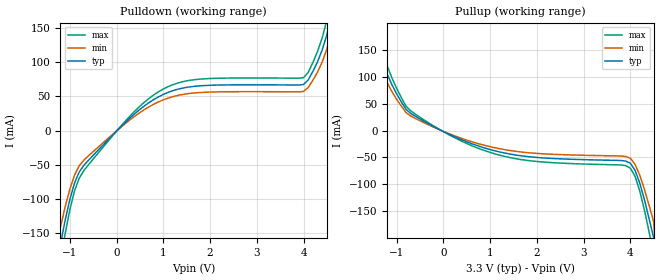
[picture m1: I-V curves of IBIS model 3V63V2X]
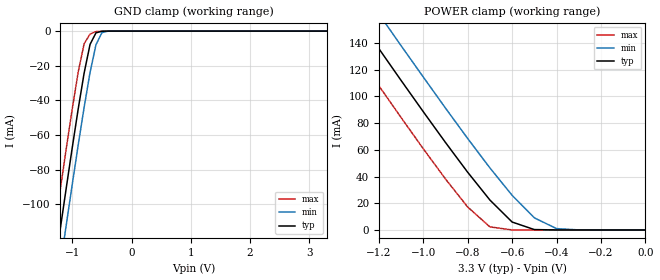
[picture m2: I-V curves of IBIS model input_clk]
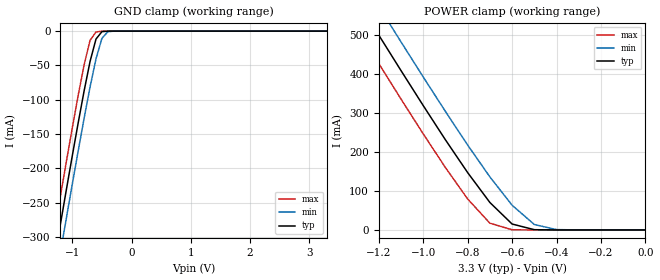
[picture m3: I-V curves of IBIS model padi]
[IBIS Ver]   2.1
[File name]   ics570-3.ibs
[File Rev]   3.0
[Date]   08/02/2010
[Source]   ICS MicroClock Applications Engineering 2
[Disclaimer] This information is for modeling purposes only, and is
(C) Copyright Integrated Circuit Systems, Inc. 1997-2001
   All rights reserved
ICS hereby grants the user of this IBIS model a non-exclusive,
nontransferable license to use this IBIS model under the following terms.
Before using this IBIS model, the user should read this license.
If the user does not accept these terms,  the IBIS model should be
returned to ICS within 30 days.
   The user is granted this license only to use the IBIS model and
is not granted rights to sell, load, rent, lease or license the IBIS
model in whole or in part, or in modified form to anyone other than
user. User may modify the IBIS model to suit its specific
applications but rights to derivative works and such modifications
shall belong to ICS.
   This IBIS model is provided on an "AS IS" basis and ICS makes
absolutely no warranty with respect to the information contained
herein. ICS DISCLAIMS AND CUSTOMER WAIVES ALL WARRANTIES, EXPRESS
OR IMPLIED, INCLUDING WARRANTIES OF MERCHANTABILITY OR FITNESS FOR
A PARTICULAR PURPOSE. The entire risk as to quality and performance
is with the Customer. ACCORDINGLY, IN NO EVENT SHALL THE COMPANY BE
LIABLE FOR ANY DAMAGES, WHETHER IN CONTRACT OR TORT,INCLUDING ANY
LOST PROFITS OR OTHER INCIDENTAL, CONSEQUENTIAL, EXEMPLARY, OR
PUNITIVE DAMAGES ARISING OUT OF THE USE OR APPLICATION OF THE IBIS
model provided in this package. Further, ICS reserves the right to
make changes without notice to any product herein to improve
reliability, function, or design. ICS does not convey any license
under patent rights or any other intellectual property rights,
including those of third parties.
   ICS is not obligated to provide maintenance or support
for the licensed IBIS model.
[Component]   ics570
[Manufacturer] Integrated Circuit Systems Inc.
[Package]
|   typ   min   max
R_pkg   40m   35m   45m
L_pkg   1.65nH   1.35nH   1.95nH
C_pkg   0.24pF   0.14pF   0.34pF
[pin]   signal_name   model_name   R_pin   L_pin   C_pin
4   ICLK   input_clk
5   FBIN   padi
7   CLK   3V63V2X
8   CLK/2   3V63V2X
| Models and submodels in the file (3): 3V63V2X (Output), input_clk (Input), padi (Input)
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|   ICS570 3.3V Clock Drive Model
| This model is suitable for all single output pins on the
| ICS570 FAMILY|
[Model]   3V63V2X
Model_type   Output
Polarity   Non-Inverting
|   typ   min   max
C_comp   5pF   4pF   6pF
|   typ   min   max
[Voltage range]  3.3V   3.15V   3.45V
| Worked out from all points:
|   slope of the pulldown table from 0 to 0.495 V, typ, clamps not added: 15.7 ohm
|   slope of the pullup table from 0 to 0.495 V, typ, clamps not added: 26.1 ohm
[pulldown]
|Voltage I (typ)   I (min)   I (max)
-3.3V     -3A        -3A        -3A
-1.3V     -199.9mA   -169.9mA   -229.9mA
-1.1V     -132mA     -112.2mA   -151.8mA
-900mV    -77.23mA   -65.65mA   -88.82mA
-700mV    -51.19mA   -43.51mA   -58.87mA
400mV     25.31mA    21.51mA    29.1mA
1.1V      55.9mA     47.52mA    64.28mA
4V        67.53mA    57.4mA     77.66mA
4.5V      140.8mA    119.7mA    161.9mA
4.6V      173.4mA    147.4mA    199.5mA
4.7V      200.4mA    170.3mA    230.4mA
6.6V      3A         3A         3A
[pullup]
|Voltage I (typ)   I (min)   I (max)
-3.3V     3A         3A         3A
-1.5V     200.3mA    170.3mA    230.4mA
-1.4V     161.7mA    137.4mA    185.9mA
-1.2V     103.9mA    88.33mA    119.5mA
-800mV    39.29mA    33.4mA     45.19mA
200mV     -10.06mA   -8.55mA    -11.57mA
1.6V      -46.18mA   -39.25mA   -53.1mA
4V        -60.82mA   -51.69mA   -69.94mA
4.2V      -97.59mA   -82.95mA   -112.2mA
4.4V      -163.8mA   -139.2mA   -188.4mA
4.5V      -199.9mA   -169.9mA   -229.9mA
6.6V      -3A        -3A        -3A
[Ramp]
|   typ   min   max
dV/dt_r   1.68/0.51n   1.60/0.56n   1.76/0.46n
dV/dt_f   1.78/0.42n   1.69/0.46n   1.87/0.38n
|   Model input_clk
[Model]   input_clk
Model_type   Input
Vinl =  0.650000V
Vinh =  2.650000V
C_comp   5.50000pF   5.00000pF   6.00000pF
[Temperature Range]   25.00000   85.00000   -40.00000
[Voltage Range]   3.30000V   3.13500V   3.46500V
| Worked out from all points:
|   GND clamp passes 1 mA (typ) near -0.60 V on its own axis
|   POWER clamp passes 1 mA (typ) near -0.51 V on its own axis
[GND_clamp]
| voltage   I(typ)   I(min)   I(max)
-3.3V     -627mA     -647.3mA   -605.4mA
-1.3V     -137.3mA   -158.7mA   -114.5mA
-1.2V     -113.6mA   -135mA     -90.81mA
-1.1V     -90.17mA   -111.5mA   -67.44mA
-1V       -67.16mA   -88.39mA   -44.75mA
-900mV    -44.9mA    -65.74mA   -23.57mA
-800mV    -24.18mA   -43.94mA   -7.252mA
-700mV    -7.641mA   -23.82mA   -1.689mA
-600mV    -985.6uA   -7.813mA   -261.8uA
-500mV    -91.34uA   -894.2uA   -15.6uA
-400mV    -5.527uA   -54.5uA    -502.6nA
3.3V      8.251uA    8.819uA    8.25uA
[POWER_clamp]
| voltage   I(typ)   I(min)   I(max)
-3.3V     651mA      675.6mA    624mA
-1.4V     183.8mA    209.8mA    156.1mA
-1.3V     159.8mA    185.7mA    131.9mA
-1.2V     135.8mA    161.8mA    108mA
-1.1V     112mA      138mA      84.22mA
-900mV    65.51mA    91.24mA    38.21mA
-800mV    43.2mA     68.45mA    17.2mA
-700mV    22.42mA    46.47mA    2.319mA
-600mV    5.953mA    25.95mA    35.27uA
-500mV    301.9uA    9.084mA    10.09uA
-400mV    15.47uA    1.015mA    9.669uA
0V        8.236uA    7.839uA    8.664uA
|   MODEL padi
[Model]   padi
Model_type   Input
Vinh=2.65V
Vinl=0.65V
C_comp   5.5pF   5.0pF   6.0pF
[Voltage range]   3.3   3.0   3.6
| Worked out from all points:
|   GND clamp passes 1 mA (typ) near -0.50 V on its own axis
|   POWER clamp passes 1 mA (typ) near -0.50 V on its own axis
[GND_clamp]
|  Voltage   I(typ)   I(min)   I(max)
-3.3V     -1.37A     -1.409A    -1.331A
-1.3V     -331.8mA   -373.2mA   -290.8mA
-1.2V     -281.3mA   -322.7mA   -240.2mA
-1.1V     -231.2mA   -272.6mA   -190.2mA
-900mV    -133.5mA   -174.4mA   -93.39mA
-800mV    -86.94mA   -126.8mA   -48.84mA
-700mV    -44.15mA   -81.44mA   -13.49mA
-600mV    -11.56mA   -40.46mA   -1.257mA
-500mV    -795uA     -10.56mA   -77.54uA
-400mV    -27.71uA   -852.7uA   -1.223uA
3.3V      227.9pA    44.02uA    159.3pA
[POWER_clamp]
|  Voltage   I(typ)   I(min)   I(max)
-3.3V     2.484A     2.554A     2.415A
-1.3V     592.5mA    666.2mA    519.5mA
-1.2V     500.5mA    574.3mA    427.4mA
-1.1V     409.4mA    483.1mA    336.3mA
-900mV    231.5mA    304.4mA    160.2mA
-800mV    147.3mA    218.1mA    79.55mA
-700mV    70.56mA    136.3mA    17.43mA
-600mV    15.25mA    63.53mA    531.6uA
-500mV    728.2uA    14mA       8.075uA
-400mV    20.89uA    955uA      118.3nA
0V        227.9pA    10.63nA    207.3pA
